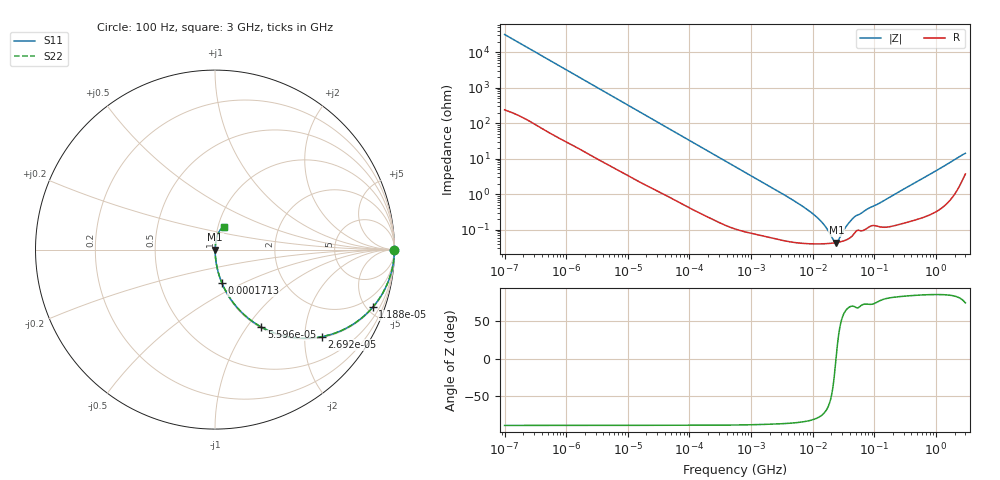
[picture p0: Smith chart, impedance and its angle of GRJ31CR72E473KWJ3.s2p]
!Murata Part Number: GRJ31CR72E473KWJ3
!These Parameters are Measured in Series Mode Connection
!Data Generated on Jun 19, 2026
!  o--ll--o
!Port1  Port2
!  o------o
!Operation Temp=25[degC], DC Bias Voltage=0[V]
!Freq. Start=100[Hz] Stop=3[GHz] 401[Steps]
# Hz S RI R 50
!Freq.(Hz) S11(Real) S11(Imag) S21(Real) S21(Imag) S12(Real) S12(Imag) S22(Real) S22(Imag)
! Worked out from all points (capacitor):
!   401 points, 100 Hz to 3 GHz, reference 50 ohm
!   read as one part in series: C = 50.4 nF near 109 Hz
!   lowest |Z| = 43.9 mohm at 24.18 MHz (marker M1)
!   series resonance near 23.88 MHz, so ESL is about 880 pH
!   S11 on the Smith chart (normalised r, x): 100 Hz: open; 11.88 kHz: 1.06, -5.47; 26.92 kHz: 1.03, -2.43; 55.95 kHz: 1.01, -1.17; 171.3 kHz: 1.01, -0.39; 3 GHz: 1.07, +0.28
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100  1 -0.00317  3.4e-05 0.00317  3.4e-05 0.00317  1 -0.00317
1788  0.9964 -0.0554  0.00362 0.0554  0.00362 0.0554  0.9964 -0.0554
4812  0.9769 -0.1453  0.0231 0.1453  0.0231 0.1453  0.9769 -0.1453
11882  0.8795 -0.3203  0.1205 0.3203  0.1205 0.3203  0.8795 -0.3203
17504  0.7736 -0.4132  0.2264 0.4132  0.2264 0.4132  0.7736 -0.4132
26919  0.5946 -0.4854  0.4054 0.4854  0.4054 0.4854  0.5946 -0.4854
31977  0.5113 -0.4941  0.4887 0.4941  0.4887 0.4941  0.5113 -0.4941
55955  0.2589 -0.4321  0.7411 0.4321  0.7411 0.4321  0.2589 -0.4321
93790  0.1131 -0.3105  0.8869 0.3105  0.8869 0.3105  0.1131 -0.3105
171338  0.0383 -0.1854  0.9617 0.1854  0.9617 0.1854  0.0383 -0.1854
547723  0.00474 -0.0606  0.9953 0.0606  0.9953 0.0606  0.00474 -0.0606
4141163  0.000528 -0.00797  0.9995 0.00797  0.9995 0.00797  0.000528 -0.00797
9794414  0.000411 -0.0029  0.9996 0.0029  0.9996 0.0029  0.000411 -0.0029
1.442825e7  0.000406 -0.00151  0.9996 0.00151  0.9996 0.00151  0.000406 -0.00151
2.12544e7  0.000424 -0.000336  0.9996 0.000336  0.9996 0.000336  0.000424 -0.000336
2.418395e7  0.000438 3.65e-05  0.9996 -3.65e-05  0.9996 -3.65e-05  0.000438 3.65e-05
2.635803e7  0.00045 0.000286  0.9996 -0.000286  0.9996 -0.000286  0.00045 0.000286
3.562563e7  0.000529 0.0012  0.9995 -0.0012  0.9995 -0.0012  0.000529 0.0012
4.612319e7  0.000751 0.00207  0.9992 -0.00207  0.9992 -0.00207  0.000751 0.00207
1.751444e8  0.00128 0.00813  0.9987 -0.00813  0.9987 -0.00813  0.00128 0.00813
8.989236e8  0.00459 0.0409  0.9954 -0.0409  0.9954 -0.0409  0.00459 0.0409
3e9  0.0527 0.1256  0.9473 -0.1256  0.9473 -0.1256  0.0527 0.1256
